(* Logix 5000 Rung export; software revision 16.03 *)

MODULES
   PDPMV1_60 : vendor None type None code None
   Local : vendor None type None code None
END_MODULES

TYPE PDPMV1_ModuleDef :   // Main module definition
STRUCT
   Output : SINT[1536];   // Output data
   Input : SINT[1536];   // Input data
   BP : PDPMV1_backplane2;   // Backplane status
   Status : PDPMV1_Status;   // Module status information
   MailboxCommand : PDPMV1_Command;   // Mailbox Command
   Mailbox : PDPMV1_Mailbox;   // Mailbox tags for optional applications
   CRC : PDPMV1_CRC_Struct;   // CRC status
   MailboxControl : PDPMV1_MBControl;   // Mailbox Control
   Util : PDPMV1_Util;   // Internal tags used for ladder logic processing. User applications should not overwrite any Util tags
END_STRUCT
END_TYPE

TYPE PDPMV1_Class1AcyclicRead_In :   // DPV1 acyclic read mailbox response
STRUCT
   ByteCount : INT;   // Byte count data block
   SlotNumber : SINT;   // Used in the slave to address the desired data block.
   SlaveAddress : SINT;   // Destination of slave (1-125)
   Length : SINT;   // Specifies the number of bytes of the data block to read
   Index : SINT;   // Index block
   ErrorDecode : SINT;   // If other than 0, refer to user manual for code information
   ErrorCode2 : SINT;   // If other than 0, refer to user manual for code information
   ErrorCode1 : SINT;   // If other than 0, refer to user manual for code information
   ExtendedFaultInfo : SINT;   // If other than 0, refer to user manual for code information
   FaultInformation : SINT;   // If other than 0, refer to user manual for code information
   Data : SINT[300];   // Returned data [1...n] array
END_STRUCT
END_TYPE

TYPE PDPMV1_GetSlaveConfig_In :   // GetSlaveConfig mailbox response
STRUCT
   ByteCount : INT;   // Byte count data block
   WordCount : INT;   // Word count data block
   SlaveAddress : INT;   // Destination of slave (1-125)
   ErrorCode : INT[1];   // If other than 0, refer to user manual for code information
   ReturnCode : INT;   // If other than 0, refer to user manual for code information
   FaultInformation : INT;   // If other than 0, refer to user manual for code information
   Identifier : SINT[245];   // Configuration from a specific connected PROFIBUS slave
END_STRUCT
END_TYPE

TYPE PDPMV1_backplane :   // This object stores variables used by the sample ladder for handshaking.
STRUCT
   Read : INT;   // Backplane read statistics
   Write : INT;   // Backplane write statistics
   Error : INT;   // Backplane error statistics
   LastRead : INT;   // Last read block index received from the module
   LastWrite : INT;   // Last write block index received from the module
   BlockIndex : INT;   // Block index of each copy of PROFIBUS input and output blocks
END_STRUCT
END_TYPE

TYPE PDPMV1_Status :   // Status block 0 or -1 for the MVI56-PDPMV1 module
STRUCT
   Pattern : SINT[12];   // Module indentification code
   Input_Size : INT;   // Input data size
   Output_Size : INT;   // Output data size
   Reserved_16 : INT;   // Reserved
   Reserved_18 : INT;   // Reserved
   Reserved_20 : INT;   // Reserved
   Input_Swap : SINT;   // User configured flag to indicate if input data is swapped before placing in the input image of the controller
   Output_Swap : SINT;   // User configured flag to indicate if output data is swapped before placing in the output image of the controller
   Module_Major_Ver : SINT;   // Module software major version number
   Module_Minor_Ver : SINT;   // Module software minor version number
   Fieldbus : PDPMV1_Fieldbus;   // PROFIBUS network status information
   Control : PDPMV1_Control;   // Module information
   Profibus_CRC32 : DINT;   // Profibus CRC32 value
   Module_CRC32 : DINT;   // Module CRC32 value
   Module : PDPMV1_Module;   // General module status to monitor data, mailbox and alarm exchange between the processor and the module
   Backplane : PDPMV1_backplane;   // Backplane status information
   Other : PDPMV1_other_status;   // General mailbox and cfg error information
END_STRUCT
END_TYPE

TYPE PDPMV1_Control :   // Control status
STRUCT
   serial_number : SINT[4];   // Module serial number
   version_MSB : SINT;   // Module version number (most significant byte)
   version_LSB : SINT;   // Module version number (least significant byte)
   mod_status_MSB : SINT;   // Module status (most significant byte)
   mod_status_LSB : SINT;   // Module status (least significant byte)
END_STRUCT
END_TYPE

TYPE PDPMV1_CRC_Struct :   // Module CRC structures
STRUCT
   In : PDPMV1_CRC;   // Mailbox response
   Out : PDPMV1_CRC;   // Mailbox request
END_STRUCT
END_TYPE

TYPE PDPMV1_Util :
STRUCT
   ByteSwapUtil : INT;   // Used for byte swap logic
   TempInt : INT;   // Used for integer formatting
   UtilCount : INT;   // Used for util count range
   Finishmailboxreading : BOOL;   // Used to finish mailbox requests and response reading
   TempInt2 : INT;   // Used to copy value to it then use it for comparison
   SetSlaveAddress101 : BOOL;   // Change the slave's PROFIBUS address 101 (only if slave supports this feature)
   SetSlaveAddress102 : BOOL;   // Change the slave's PROFIBUS address 102 (only if slave supports this feature)
   Class1AcyclicWrite101 : BOOL;   // Request the module to send acyclic write message to the slave
   Class1AcyclicWrite102 : BOOL;   // Request the module to send acyclic write message to the slave
   Class2AcyclicWrite101 : BOOL;   // Request the module to send Class2 acyclic write message to slave 101
   Class2AcyclicWrite102 : BOOL;   // Request the module to send Class2 acyclic write message to slave 102
   Finishgetlivelist : BOOL;   // Finish requesting the Live List information from the module
   FinishgetSlaveconfig : BOOL;   // Finish requesting configuration information from a slave
   FinishgetSlaveDiagnost : BOOL;   // Finish requesting slave diagnostics from a slave
   FinishSetSlaveAddr : BOOL;   // Finish changing the slaves PROFIBUS addressing
   FinishClass1AcyclicRead : BOOL;   // Finish requesting the module to send acyclic read message to slave
   FinishClass1AcyclicWrite : BOOL;   // Finish requesting the module to send acyclic write message to slave
   FinishStartStopSlaves : BOOL;   // Finish PROFIBUS communications with one or more slaves if supported
   FinishClass2AcyclicRead : BOOL;   // Finish requesting the module to send Class 2 acyclic read message to slave
   FinishClass2AcyclicWrite : BOOL;   // Finish requesting the module to send acyclic write message to slave
END_STRUCT
END_TYPE

TYPE PDPMV1_Class1AcyclicWrite_Out :   // DPV1 acyclic write mailbox request
STRUCT
   SlotNumber : SINT;   // Used in the slave to address the desired data block.
   SlaveAddress : SINT;   // Destination of slave (1-125)
   DataSize : INT;   // Object data size
   Length : SINT;   // Specifies the number of bytes of the data block to read
   Index : SINT;   // Index Block
   Data : SINT[300];   // Data that should be written [1...n]
END_STRUCT
END_TYPE

TYPE PDPMV1_AbortConnection_out :
STRUCT
   C_REF : INT;   // Connection reference that shall be terminated
   ReasonCode : SINT;   // Indicates the reason for the abort request. Value is user-specific. Range 0...15.
   Subnet : SINT;   // This parameter encodes information about the origin of the abort initiator. 0: No 1: Local 2: Remote
END_STRUCT
END_TYPE

TYPE PDPMV1_Class1AcyclicWrite_In :   // DPV1 acyclic write mailbox response
STRUCT
   ByteCount : INT;   // Byte count data block
   SlotNumber : SINT;   // Used in the slave to address the desired data block.
   SlaveAddress : SINT;   // Destination of slave (1-125)
   Length : SINT;   // Specifies the number of bytes of the data block to read
   Index : SINT;   // Index block
   ErrorDecode : SINT;   // If other than 0, refer to user manual for code information
   ErrorCode2 : SINT;   // If other than 0, refer to user manual for code information
   ErrorCode1 : SINT;   // If other than 0, refer to user manual for code information
   ExtendedFaultInfo : INT;   // If other than 0, refer to user manual for code information
   FaultInformation : INT;   // If other than 0, refer to user manual for code information
   Data : SINT[300];   // Returned data [1...n] array
END_STRUCT
END_TYPE

TYPE PDPMV1_GetSlaveConfig :   // GetSlaveConfig mailobox to retrieve configuration data from specific PROFIBUS slaves
STRUCT
   Out : PDPMV1_GetSlaveConfig_Out;   // mailbox request
   In : PDPMV1_GetSlaveConfig_In;   // mailbox response
END_STRUCT
END_TYPE

TYPE PDPMV1_Class2AcyclicRead_In :
STRUCT
   DataSize : INT;   // Byte count data block
   C_REF : INT;   // Connections references used to identify the connection later on. Range: 1-128
   Index : SINT;   // Index block
   SlotNumber : SINT;   // Used in the slave to address the desired data block.
   Length : INT;   // Specifies the number of bytes of the data block to read
   ErrorDecode : INT;   // If other than 0, refer to user manual for code information
   ErrorCode2 : SINT;   // If other than 0, refer to user manual for code information
   ErrorCode1 : SINT;   // If other than 0, refer to user manual for code information
   ExtendedFaultInfo : SINT;   // If other than 0, refer to user manual for code information
   FaultInformation : SINT;   // If other than 0, refer to user manual for code information
   Data : SINT[244];   // Returned data [1...n] array
END_STRUCT
END_TYPE

TYPE PDPMV1_Class2AcyclicWrite_In :   // DPV1 acyclic write mailbox response
STRUCT
   ByteCount : INT;   // Byte count data block
   C_REF : INT;   // Connection reference that shall be Read
   Index : SINT;   // Index block
   SlotNumber : SINT;   // Used in the slave to address the desired data block.
   Length : SINT;   // Specifies the number of bytes of the data block to read
   ErrorDecode : SINT;   // If other than 0, refer to user manual for code information
   ErrorCode2 : SINT;   // If other than 0, refer to user manual for code information
   ErrorCode1 : SINT;   // If other than 0, refer to user manual for code information
   ExtendedFaultInfo : SINT;   // If other than 0, refer to user manual for code information
   FaultInformation : SINT;   // If other than 0, refer to user manual for code information
   Data : SINT[244];   // Returned data [1...n] array
END_STRUCT
END_TYPE

TYPE PDPMV1_Module :   // Status data
STRUCT
   Mod_scan_count : INT;   // Incremented every module scan loop
   Mod_output_update : INT;   // Incremented at every output scan
   Mod_input_update : INT;   // Incremented at every input scan
   Mod_out_MB : INT;   // Incremented at every output mailbox processing
   Mod_in_MB : INT;   // Incremented at every intput mailbox processing
   Mod_alarm_ind : INT;   // Incremented at every alarm indication
   Mod_alarm_con : INT;   // Incremented at every alarm confirmation
   Reserved1 : INT;   // Reserved
   Reserved2 : INT;   // Reserved
END_STRUCT
END_TYPE

TYPE PDPMV1_Class1AcyclicRead :   // DPV1 acyclic read mailbox data structure
STRUCT
   Out : PDPMV1_Class1AcyclicRead_Out;   // Mailbox request
   In : PDPMV1_Class1AcyclicRead_In;   // Mailbox response
END_STRUCT
END_TYPE

TYPE PDPMV1_SetSlaveMode :   // SetSlaveMode mailbox that allows the processor to change the slave mode to interrupt input or output data update
STRUCT
   Out : PDPMV1_SetSlaveMode_Out;   // Mailbox Request
   In : PDPMV1_SetSlaveMode_In;   // Mailbox Response
END_STRUCT
END_TYPE

TYPE PDPMV1_GetSlaveDiagnostics_In :   // GetSlaveDiagnostics mailbox response
STRUCT
   RequestType : SINT;   // Type of request. 0 to use module memory RAM or 1 for live PROFIBUS network.
   SlaveAddress : SINT;   // Destination of slave (Range 1-125)
   ExtendedFaultInfo : INT;   // If other than 0, refer to user manual for code information
   FaultInformation : INT;   // If other than 0, refer to user manual for code information
   StationStatus1_2 : INT;   // Status of station types 1 and 2
   StationStatus3_4 : INT;   // Status of station types 3 and 4
   IdentNumber : INT;   // Unique ID assigned by the PROFIBUS User Organization
   ExtendedDiagnosticData : INT[200];   // Slave user-specific data. Refer to actual slave documentation for info
END_STRUCT
END_TYPE

TYPE PDPMV1_backplane2 :   // This object stores variables used by the sample ladder for handshaking.
STRUCT
   LastRead : INT;   // Last read block index received from the module
   LastWrite : INT;   // Last write block index received from the module
   BlockIndex : INT;   // Block index of each copy of PROFIBUS input and output blocks
END_STRUCT
END_TYPE

TYPE PDPMV1_Command :   // This object contains the command bits that request mailbox messages from the module.
STRUCT
   StopMode : BOOL;   // Set the module to stop mode (PROFIBUS communication is interrupted in stop mode)
   OperateMode : BOOL;   // Set the module to operate mode (module only communicates through PROFIBUS)
   ClearMode : BOOL;   // Set the module to clear mode (outputs are disabled)
   SynchCRC : BOOL;   // CRC synchronization
   GetLiveList : BOOL;   // Request the Live List information from the module
   GetSlaveConfig : BOOL;   // Request configuration information from slave
   SetSlaveMode : BOOL;   // Set the module to stop mode (PROFIBUS communication is interrupted in stop mode)
   GetSlaveDiagnostics : BOOL;   // Requests slave diagnostics from a slave
   SetSlaveAddress : BOOL;   // Change the slave's PROFIBUS address 100 (only if slave supports this feature)
   StartSlaves : BOOL;   // Restarts PROFIBUS communication with one or more slaves after a "StopSlave" mailbox
   StopSlaves : BOOL;   // Stop PROFIBUS communication with one or more slaves
   Class1AcyclicRead : BOOL;   // Request the module to send acyclic read message to slave
   Class1AcyclicWrite : BOOL;   // Request the module to send acyclic write message to the slave
   InitiateConnection : BOOL;   // Request to establish connection with a V1 slave that can handle class 2 messages
   AbortConnection : BOOL;   // Request to Abort an already established connection with a V1 slave that can handle class 2 messages
   Class2AcyclicRead : BOOL;   // Request the module to send class 2 acyclic Read message to a V1 slave
   Class2AcyclicWrite : BOOL;   // Request the module to send class 2 acyclic Write message to a V1 slave
END_STRUCT
END_TYPE

TYPE PDPMV1_SetSlaveMode_Out :   // Mailbox Request
STRUCT
   GroupSelect : SINT;   // Range 01h to FFh (Bit Coded). This parameter determines which group to address. Refer to the user manual for examples
   SlaveAddress : SINT;   // Range 1 to 125; 127 (Multicast address).
   ControlCommand : PDPMV1_ControlCommand;   // This parameter specifies the command to send (Unsync/Sync and Unfreeze/Freeze).
END_STRUCT
END_TYPE

TYPE PDPMV1_Fieldbus :   // Fieldbus status
STRUCT
   FB_Slave_Cfg_List : SINT[16];   // Bitmap structure containing PROFIBUS slave configuration (bit x = 1 means slave x is configured)
   FB_Slave_Data_xfer : SINT[16];   // Bitmap structure containing PROFIBUS slave data exchange status (bit x = 1 means slave x is transferring data to the module)
   FB_Slave_Diag : SINT[16];   // Bitmap structure containing PROFIBUS slave diagnostic info (bit x = 1 means slave x is reporting diagnostics)
   FB_Pad_Byte : SINT;   // Reserved
   FB_op_state : SINT;   // Operation state ( 00 = offline, 40 = stop, 80 = clear, C0= operate)
   FB_ident_MSB : SINT;   // Master identification code (most significant byte)
   FB_ident_LSB : SINT;   // Master identification code (least significant byte)
END_STRUCT
END_TYPE

TYPE PDPMV1_InitiateConnection_out :
STRUCT
   SlaveAddress : INT;   // Address of the slave to which a connection shall be established. Range: 0...126
   C_REF : INT;   // Connections references used to identify the connection later on. Range: 1-128
END_STRUCT
END_TYPE

TYPE PDPMV1_SetSlaveMode_In :   // Mailbox response
STRUCT
   GroupSelect : SINT;   // Range 01h to FFh (Bit Coded). This parameter determines which group to address. Refer to the user manual for examples
   SlaveAddress : SINT;   // Range 1 to 125; 127 (Multicast address).
   ControlCommand : PDPMV1_ControlCommand;   // This parameter specifies the command to send (Unsync/Sync and Unfreeze/Freeze).
   ExtendedFaultInfo : INT;   // If other than 0, refer to user manual for code information
   FaultInformation : INT;   // If other than 0, refer to user manual for code information
END_STRUCT
END_TYPE

TYPE PDPMV1_GetSlaveDiagnostics_Out :   // GetSlaveDiagnostics mailbox request
STRUCT
   RequestType : SINT;   // Type of request. 0 to use module memory RAM or 1 for live PROFIBUS network.
   SlaveAddress : SINT;   // Destination of slave (Range 1-125)
END_STRUCT
END_TYPE

TYPE PDPMV1_Class1AcyclicRead_Out :   // DPV1 acyclic read mailbox request
STRUCT
   SlotNumber : SINT;   // Used in the slave to address the desired data block.
   SlaveAddress : SINT;   // Destination of slave (1-125)
   DataSize : INT;   // Object data size
   Length : SINT;   // Specifies the number of bytes of the data block to read
   Index : SINT;   // Index block
END_STRUCT
END_TYPE

TYPE PDPMV1_Start_Stop_Slaves_Out :   // Mailbox request
STRUCT
   SlaveNumber : SINT[126];   // Slave number designation (1-125)
END_STRUCT
END_TYPE

TYPE PDPMV1_SetSlaveAddress :   // SetSlaveAddress mailbox that allows the module to dynamically change a PRIDUBUS address (only for slaves that supports it)
STRUCT
   Out : PDPMV1_SetSlaveAddress_Out;   // Mailbox request
   In : PDPMV1_SetSlaveAddress_In;   // Mailbox response
END_STRUCT
END_TYPE

TYPE PDPMV1_GetSlaveDiagnostics :   // GetSlaveDiagnostics mailbox to retrieve diagnostic information from specific PROFIBUS slaves
STRUCT
   Out : PDPMV1_GetSlaveDiagnostics_Out;   // Mailbox request
   In : PDPMV1_GetSlaveDiagnostics_In;   // Mailbox response
END_STRUCT
END_TYPE

TYPE PDPMV1_ControlCommand :   // Option bits for SetSlaveMode mailbox
STRUCT
   Reserved1 : BOOL;   // Reserved
   Reserved2 : BOOL;   // Reserved
   Unfreeze_Input : BOOL;   // Freeze mode is concluded when initiated
   Freeze_Input : BOOL;   // Causes the addressed slave to assume freeze mode.
   Unsynchronize_Output : BOOL;   // Unsynchronized output data
   Synchronize_Output : BOOL;   // Synchronized output data
   Reserved3 : BOOL[32];   // Reserved
END_STRUCT
END_TYPE

TYPE PDPMV1_Mailbox :   // Stores all mailbox request and response registers
STRUCT
   GetLiveList : PDPMV1_GetLiveList;   // Gets information from all nodes on the network
   GetSlaveConfig : PDPMV1_GetSlaveConfig;   // Get slave configuration
   SetSlaveMode : PDPMV1_SetSlaveMode;   // Send special control command to one or several slaves (Sync/Freeze)
   GetSlaveDiagnostics : PDPMV1_GetSlaveDiagnostics;   // Get diagnostic information from a slave
   SetSlaveAddress : PDPMV1_SetSlaveAddress;   // Set node address of a slave (if supported by the slave)
   StartStopSlaves : PDPMV1_Start_Stop_Slaves;   // Start/Stop slaves dynamically
   Class1AcyclicRead : PDPMV1_Class1AcyclicRead;   // Initiates a DPV1 class 1 acyclic read request.
   Class1AcyclicWrite : PDPMV1_Class1AcyclicWrite;   // Initiates a DPV1 class 1 acyclic write request.
   Alarm : PDPMV1_Alarm;   // Alarm message transferred by a slave to the master
   InitiateConnection : PDPMV1_InitiateConnection;   // mailbox form used to initiate connection with v1 slave before sending class2 messages.
   AbortConnection : PDPMV1_AbortConnection;   // mailbox form used to abort an already established connection with v1 slave before sending class2 messages.
   Class2AcyclicRead : PDPMV1_Class2AcyclicRead;   // mailbox form used to send a class 2 messages to read acyclic data
   Class2AcyclicWrite : PDPMV1_Class2AcyclicWrite;   // mailbox form used to send a class 2 messages to write acyclic data
END_STRUCT
END_TYPE

TYPE PDPMV1_Alarm :   // DPV1 alarm data received by the module
STRUCT
   ByteCount : INT;   // Byte count data block
   SlotNumber : SINT;   // Used in the slave to address the desired data block. Range 0-254
   SlaveAddress : SINT;   // Destination of slave (1-125)
   AlarmSpecAck : SINT;   // Additional alarm information
   SeqNumber : SINT;   // Unique ID number of the alarm. Range 0-31.
   ExtDiag : SINT;   // Extended Diagnostic Flag (FFh - flag set and 00h - flag cleared).
   AlarmType : SINT;   // Identifies alarm type. Range is from 1 to 6, 32 to 126.
   FaultInformation : SINT;   // If other than 0, refer to user manual for code information
   Data : SINT[500];   // Returned data [1...n] array with additional manf. spec alarm info.
END_STRUCT
END_TYPE

TYPE PDPMV1_GetSlaveConfig_Out :   // GetSlaveConfig mailbox request
STRUCT
   SlaveAddress : INT;   // Destination of slave (1-125)
END_STRUCT
END_TYPE

TYPE PDPMV1_Class2AcyclicRead_Out :
STRUCT
   C_REF : INT;   // Connection reference that shall be terminated
   Index : SINT;   // Used in the slave for addressing of the desired data block. Range 0...254
   SlotNumber : SINT;   // Used in the slave for addressing of the desired data block. Range 0...254
   Length : INT;   // Number of bytes to write
END_STRUCT
END_TYPE

TYPE PDPMV1_GetLiveList :   // GetLiveList mailbox to retrieve the live list information from PROFIBUS network, informing the slaves that are communicating
STRUCT
   ReturnCode : SINT;   // Returned code about the nodes on the network
   FaultInfo : SINT;   // If other than 0, refer to user manual for code information
   Station : SINT[127];   // Station type contents.
END_STRUCT
END_TYPE

TYPE PDPMV1_AbortConnection_In :
STRUCT
   C_REF : INT;   // Connection reference that shall be terminated.
   ReasonCode : SINT;   // Indicates the reason for the abort request. Value is user-specific. Range 0...15
   Subnet : SINT;   // This parameter encodes information about the origin of the abort initiator. 0: No 1: Local 2: Remote 3...255: (reserved)
   ExtendedFaultInformation : INT;   // If ‘Fault Information’ equals 000Ah or 000Bh, additional information of the error can be found here. For more information,
   FaultInformation : INT;   // If ‘Invalid Other’ is returned in the Message Information word in the header of the response,
END_STRUCT
END_TYPE

TYPE PDPMV1_CRC :   // This object stores CRC values for both Profibus and the module.
STRUCT
   ProfibusCRC : DINT;   // Stores Profibus CRC32 values
   ModuleCRC : DINT;   // Stores Module CRC32 values
END_STRUCT
END_TYPE

TYPE PDPMV1_SetSlaveAddress_Out :   // Mailbox request
STRUCT
   ByteCount : INT;   // Byte count data block
   NewSlaveAddress : SINT;   // Range 1 to 125, specifies the new address of the slave
   CurrentSlaveAddress : SINT;   // Range 1 to 125, specifies the current address of the slave
   SlaveIdentNumber : INT;   // Indent number for the slave
   No_add_Chg : INT;   // specifies whether it is allowed to change the slave address again later
   MessageDataByte : SINT[400];   // Message data byte array for user-specific data
END_STRUCT
END_TYPE

TYPE PDPMV1_InitiateConnection :
STRUCT
   Out : PDPMV1_InitiateConnection_out;   // Mailbox Request
   In : PDPMV1_InitiateConnection_In;   // Mailbox response
END_STRUCT
END_TYPE

TYPE PDPMV1_Class2AcyclicWrite_Out :   // DPV1 acyclic write mailbox request
STRUCT
   DataSize : INT;   // Object data size
   C_REF : INT;   // Connection reference that shall be terminated
   Index : SINT;   // Index block
   SlotNumber : SINT;   // Used in the slave to address the desired data block.
   Length : INT;   // Specifies the number of bytes of the data block to read
   Data : SINT[244];   // Data that should be written [1...n]
END_STRUCT
END_TYPE

TYPE PDPMV1_other_status :   // This object contains specific information, such as the number of mailbox and alarms located in the mailbox queue.
STRUCT
   Cfg_file_error : INT;   // Bit0 = PDPMV1.CFG, Bit 1 = WATTCP.CFG, Bit 2 = PDPMV1.DDB, Bit3=PDPMV1.XML
   R_120 : INT;   // Not Used
   R_122 : INT;   // Not Used
   R_124 : INT;   // Not Used
   R_126 : INT;   // Not Used
   R_128 : INT;   // Not Used
   R_130 : INT;   // Not Used
   R_132 : INT;   // Not Used
   R_134 : INT;   // Not Used
   R_136 : INT;   // Not Used
   R_138 : INT;   // Not Used
   R_140 : INT;   // Not Used
   R_142 : INT;   // Not Used
   R_144 : INT;   // Not Used
   In_MB_queue : INT;   // Number of messages in the input mailbox queue
   Out_MB_queue : INT;   // Number of messages in the output mailbox queue
   Alarm_MB_queue : INT;   // Number of messages in the alarm mailbox queue
   Last_out_MB : INT;   // Number of messages in the output mailbox queue
   Cur_in_MB : INT;   // Number of messages currently in the input mailbox queue
   Cur_alarm_MB : INT;   // Number of messages currently in the alarm mailbox queue
END_STRUCT
END_TYPE

TYPE PDPMV1_Class2AcyclicWrite :   // DPV1 acyclic write mailbox data structure
STRUCT
   Out : PDPMV1_Class2AcyclicWrite_Out;   // Mailbox request
   In : PDPMV1_Class2AcyclicWrite_In;   // Mailbox response
END_STRUCT
END_TYPE

TYPE PDPMV1_Start_Stop_Slaves :   // Start/Stop Slaves mailbox allows the processor to restart or hault slave communication.
STRUCT
   Out : PDPMV1_Start_Stop_Slaves_Out;   // Mailbox Request
   In : PDPMV1_Start_Stop_Slaves_In;   // Mailbox Response
END_STRUCT
END_TYPE

TYPE PDPMV1_Class1AcyclicWrite :   // DPV1 acyclic write mailbox data structure
STRUCT
   Out : PDPMV1_Class1AcyclicWrite_Out;   // Mailbox request
   In : PDPMV1_Class1AcyclicWrite_In;   // Mailbox response
END_STRUCT
END_TYPE

TYPE PDPMV1_Class2AcyclicRead :
STRUCT
   Out : PDPMV1_Class2AcyclicRead_Out;   // Mailbox request
   In : PDPMV1_Class2AcyclicRead_In;   // Mailbox response
END_STRUCT
END_TYPE

TYPE PDPMV1_MBControl :   // PDPMV1 Mailbox Control status.
STRUCT
   Out_MB_index : INT;   // Reserved
   In_MB_index : INT;   // Reserved
   Alarm_MB_index : INT;   // Reserved
   In_Last_Out_MB : INT;   // Last out mailbox message ID processed from output image
   In_Last_In_MB : INT;   // Current in mailbox control index
   In_Last_Alarm_MB : INT;   // Current alarm control index
   Out_Last_Out_MB : INT;   // Reserved
   Out_Last_In_MB : INT;   // Reserved
   Out_Last_Alarm_MB : INT;   // Reserved
END_STRUCT
END_TYPE

TYPE PDPMV1_AbortConnection :
STRUCT
   Out : PDPMV1_AbortConnection_out;   // Mailbox Request
   In : PDPMV1_AbortConnection_In;   // Mailbox Response
END_STRUCT
END_TYPE

TYPE PDPMV1_SetSlaveAddress_In :   // Mailbox response
STRUCT
   ByteCount : INT;   // Byte count data block
   NewSlaveAddress : SINT;   // Range 1 to 125, specifies the new address of the slave
   CurrentSlaveAddress : SINT;   // Range 1 to 125, specifies the current address of the slave
   SlaveIdentNumber : INT;   // Indent number for the slave
   No_add_Chg : INT;   // specifies whether it is allowed to change the slave address again later
   ErrorCode1_2 : INT;   // If other than 0, refer to user manual for code information
   ErrorCode3_4 : INT;   // If other than 0, refer to user manual for code information
   ReturnCode : INT;   // If other than 0, refer to user manual for code information
   FaultInformation : INT;   // If other than 0, refer to user manual for code information
   MessageDataByte : SINT[400];   // Message data byte array for user-specific data
END_STRUCT
END_TYPE

TYPE PDPMV1_Start_Stop_Slaves_In :   // Mailbox response
STRUCT
   AdditionalFaultInfo : INT;   // If other than 0, refer to user manual for code information
   FaultInformation : INT;   // If other than 0, refer to user manual for code information
   SlaveNumber : SINT[126];   // Slave number designation (Range 1-125)
END_STRUCT
END_TYPE

TYPE PDPMV1_InitiateConnection_In :   // This tag holds the response parameters after the user sends mailbox to initiate connection with V1 slave
STRUCT
   SizeofdatainBytes : INT;   // Size of data being read
   C_REF : INT;   // Connections references used to identify the connection later on. Range: 1-128
   MaxDataLength : SINT;   // The slave’s maximum data length in bytes (reported by the slave in DP Initiate.res).
   SlaveAddress : SINT;   // Address of the slave to which a connection shall be established. Range: 0...126
   MinmumSlaveTimeout : INT;   // The minimum slave timeout value supported by the slave (in multiples of 10ms).
   ErrorDecode : SINT;   // If ‘Fault Information’ equals 0010h, additional information according to the DPV1 specification
   ErrorCode2 : SINT;   // If ‘Fault Information’ equals 0010h, additional information according to the DPV1 specification
   ErrorCode1 : SINT;   // If ‘Fault Information’ equals 0010h, additional information according to the DPV1 specification
   ExtendedFaultInformation : INT;   // If ‘Fault Information’ equals 000Ah or 000Bh, additional information of the error can be found here. For more information, see
   FaultInformation : INT;   // If ‘Invalid Other’ is returned in the Message Information word in the header of the response, information about the fault
   SendTimeout : INT;   // Defines the control time (timebase 10ms) for the supervision of the connection between the slave and the master. Range 6...655
   FeatureSupported2 : SINT;   // (reserved for future use)
   FeatureSupported1 : SINT;   // Identifies the supported C2-service functionality as follows: b0: DPV1_RW. This bit is set if the services C2_Read and C2_Write
   ProfileFeatures2 : SINT;   // Identifies the supported service functionality regarding the used profile definition. The meaning of these registers are profil
   ProfileFeatures1 : SINT;   // Identifies the supported service functionality regarding the used profile definition. The meaning of these registers are profil
   ProfileIdentNumber : INT;   // This parameter identifies a unique profile definition. The Profile Ident Number is taken from the pool of Ident Numbers managed
   S_Length : SINT;   // This parameter specifies the length of the S_Address parameter (see table below). Default value is 02h.
   S_Type : SINT;   // This parameter indicates the presence of the optional Network/MAC address of the source. b0: 1: A Network/MAC address is presen
   D_Length : SINT;   // This value specifies the length of the D_Address parameter (see table below). Default value is 02h.
   D_Type : SINT;   // This parameter indicates the presence of the optional Network/MAC address of the destination. b0: 1: A Network/MAC address is p
   S_Address : INT;   // This field holds additional address information about the source. It’s structure depends on the settings in S_Type.
   D_Address : INT;   // This field holds additional address information about the destination. It’s structure depends on the settings in D_Type
END_STRUCT
END_TYPE

ADD_ON_INSTRUCTION AOI69PDPMV1_60   (* revision 1.4, vendor ProSoft Technology Inc. *)
// Add-On - MVI69-PDPMV1(Block size 60).
// Revision note:
// v1.4 - Added support for class 2 messages that was supported in a specific  V1 slaves.
VAR_IN_OUT
   Connection_Input : INT[62]; {required}   // Connection Input to be associated to the MVI69PDPMV1 Input Array
   Connection_Output : INT[61]; {required}   // Connection Output to be associated to the MVI69-PDPMV1 Output Array
   MVI69PDPMV1 : PDPMV1_ModuleDef; {required}
END_VAR

ROUTINE Logic   (* ladder *)
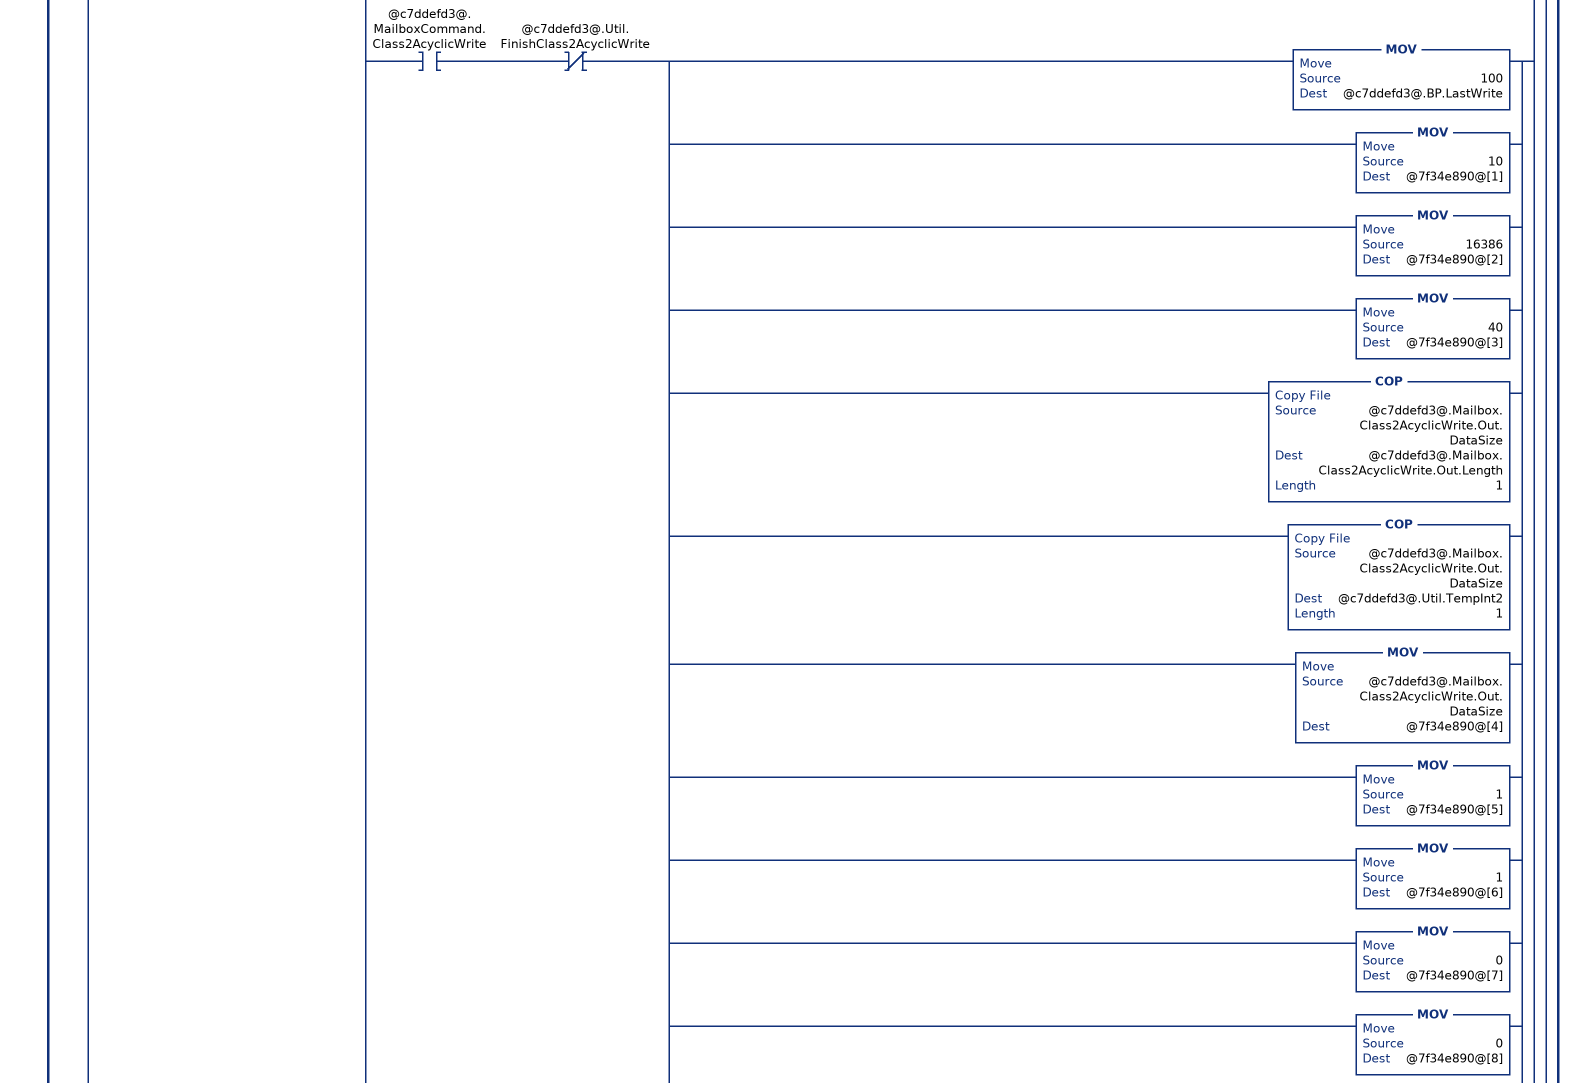
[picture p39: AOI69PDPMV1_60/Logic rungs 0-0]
   // This rung is used to verify if the module has sent a new input block to the processor. The trigger is when the input image offset 0 (Read Block ID) is different than the last one processed by the processor
   0: NEQ(@8b565331@[0],@c7ddefd3@.BP.LastRead)[MOV(@8b565331@[0],@c7ddefd3@.BP.LastRead) ,EQU(@c7ddefd3@.BP.LastRead,-1) [COP(@8b565331@[2],@c7ddefd3@.Status.Pattern[0],20) ,COP(@8b565331@[13],@c7ddefd3@.Status.Input_Swap,4) ,COP(@8b565331@[15],@c7ddefd3@.Status.Fieldbus.FB_Slave_Cfg_List[0],52) ,COP(@8b565331@[41],@c7ddefd3@.Status.Control.serial_number[0],8) ,COP(@8b565331@[45],@c7ddefd3@.Status.Profibus_CRC32,2) ] ,EQU(@c7ddefd3@.BP.LastRead,0) [COP(@8b565331@[2],@c7ddefd3@.Status.Module.Mod_scan_count,9) ,COP(@8b565331@[11],@c7ddefd3@.Status.Backplane.Read,3) ,COP(@8b565331@[14],@c7ddefd3@.Status.Other.Cfg_file_error,20) ] ,LIM(1,@c7ddefd3@.BP.LastRead,16) [LIM(1,@c7ddefd3@.BP.LastRead,15) [CPT(@c7ddefd3@.BP.BlockIndex,(@c7ddefd3@.BP.LastRead-1)*100) ,COP(@8b565331@[2],@c7ddefd3@.Input[@c7ddefd3@.BP.BlockIndex],100) ] ,EQU(@c7ddefd3@.BP.LastRead,16) COP(@8b565331@[2],@c7ddefd3@.Input[1500],36) ,COP(@8b565331@[52],@c7ddefd3@.MailboxControl.In_Last_Out_MB,2) ,COP(@8b565331@[56],@c7ddefd3@.CRC.In.ProfibusCRC,2) ] ,LIM(100,@c7ddefd3@.BP.LastRead,102) [EQU(100,@c7ddefd3@.BP.LastRead) LIM(0,@8b565331@[2],2) [OTU(@c7ddefd3@.MailboxCommand.StopMode) ,OTU(@c7ddefd3@.MailboxCommand.OperateMode) ,OTU(@c7ddefd3@.MailboxCommand.ClearMode) ,OTU(@c7ddefd3@.MailboxCommand.SetSlaveMode) ] ,XIC(@c7ddefd3@.Util.Finishgetlivelist) [EQU(@8b565331@[4],24) EQU(100,@c7ddefd3@.BP.LastRead) [MOV(@8b565331@[5],@c7ddefd3@.Util.UtilCount) ,COP(@8b565331@[18],@c7ddefd3@.Mailbox.GetLiveList.Station[0],88) ,LEQ(@c7ddefd3@.Util.UtilCount,88) OTU(@c7ddefd3@.Util.Finishgetlivelist) ] ,EQU(101,@c7ddefd3@.BP.LastRead) [COP(@8b565331@[2],@c7ddefd3@.Mailbox.GetLiveList.Station[88],39) ,OTU(@c7ddefd3@.Util.Finishgetlivelist) ] ] ,EQU(@8b565331@[4],3) [COP(@8b565331@[10],@c7ddefd3@.Mailbox.SetSlaveMode.In.GroupSelect,2) ,MOV(@8b565331@[11],@c7ddefd3@.Util.TempInt) ,SWPB(@c7ddefd3@.Util.TempInt,REVERSE,@c7ddefd3@.Util.ByteSwapUtil) ,COP(@c7ddefd3@.Util.ByteSwapUtil,@c7ddefd3@.Mailbox.SetSlaveMode.In.ControlCommand,1) ,MOV(@8b565331@[16],@c7ddefd3@.Mailbox.SetSlaveMode.In.ExtendedFaultInfo) ,MOV(@8b565331@[17],@c7ddefd3@.Mailbox.SetSlaveMode.In.FaultInformation) ] ,XIC(@c7ddefd3@.Util.FinishgetSlaveDiagnost) [EQU(100,@c7ddefd3@.BP.LastRead) EQU(@8b565331@[4],4) [MOV(@8b565331@[5],@c7ddefd3@.Util.UtilCount) ,COP(@8b565331@[10],@c7ddefd3@.Mailbox.GetSlaveDiagnostics.In.RequestType,2) ,MOV(@8b565331@[16],@c7ddefd3@.Mailbox.GetSlaveDiagnostics.In.ExtendedFaultInfo) ,MOV(@8b565331@[17],@c7ddefd3@.Mailbox.GetSlaveDiagnostics.In.FaultInformation) ,MOV(@8b565331@[18],@c7ddefd3@.Mailbox.GetSlaveDiagnostics.In.StationStatus1_2) ,MOV(@8b565331@[19],@c7ddefd3@.Mailbox.GetSlaveDiagnostics.In.StationStatus3_4) ,MOV(@8b565331@[20],@c7ddefd3@.Mailbox.GetSlaveDiagnostics.In.IdentNumber) ,COP(@8b565331@[21],@c7ddefd3@.Mailbox.GetSlaveDiagnostics.In.ExtendedDiagnosticData[0],41) ,LEQ(@c7ddefd3@.Util.UtilCount,41) OTU(@c7ddefd3@.Util.FinishgetSlaveDiagnost) ] ,EQU(101,@c7ddefd3@.BP.LastRead) [SUB(@c7ddefd3@.Util.UtilCount,41,@c7ddefd3@.Util.UtilCount) ,COP(@8b565331@[2],@c7ddefd3@.Mailbox.GetSlaveDiagnostics.In.ExtendedDiagnosticData[41],60) ,LEQ(@c7ddefd3@.Util.UtilCount,60) OTU(@c7ddefd3@.Util.FinishgetSlaveDiagnost) ] ,EQU(102,@c7ddefd3@.BP.LastRead) [COP(@8b565331@[2],@c7ddefd3@.Mailbox.GetSlaveDiagnostics.In.ExtendedDiagnosticData[101],24) ,OTU(@c7ddefd3@.Util.FinishgetSlaveDiagnost) ] ] ,XIC(@c7ddefd3@.Util.FinishgetSlaveconfig) [EQU(@c7ddefd3@.BP.LastRead,100) EQU(@8b565331@[4],5) [MOV(@8b565331@[5],@c7ddefd3@.Mailbox.GetSlaveConfig.In.ByteCount) ,MOV(@8b565331@[10],@c7ddefd3@.Util.ByteSwapUtil) ,SWPB(@c7ddefd3@.Util.ByteSwapUtil,REVERSE,@c7ddefd3@.Mailbox.GetSlaveConfig.In.SlaveAddress) ,COP(@8b565331@[14],@c7ddefd3@.Mailbox.GetSlaveConfig.In.ErrorCode[0],2) ,MOV(@8b565331@[16],@c7ddefd3@.Mailbox.GetSlaveConfig.In.ReturnCode) ,MOV(@8b565331@[17],@c7ddefd3@.Mailbox.GetSlaveConfig.In.FaultInformation) ,COP(@8b565331@[18],@c7ddefd3@.Mailbox.GetSlaveConfig.In.Identifier[0],88) ,LEQ(@c7ddefd3@.Mailbox.GetSlaveConfig.In.ByteCount,88) OTU(@c7ddefd3@.Util.FinishgetSlaveconfig) ] ,EQU(@c7ddefd3@.BP.LastRead,101) [SUB(@c7ddefd3@.Mailbox.GetSlaveConfig.In.ByteCount,88,@c7ddefd3@.Mailbox.GetSlaveConfig.In.ByteCount) ,COP(@8b565331@[2],@c7ddefd3@.Mailbox.GetSlaveConfig.In.Identifier[88],120) ,LEQ(@c7ddefd3@.Mailbox.GetSlaveConfig.In.ByteCount,120) OTU(@c7ddefd3@.Util.FinishgetSlaveconfig) ] ,EQU(@c7ddefd3@.BP.LastRead,102) [COP(@8b565331@[2],@c7ddefd3@.Mailbox.GetSlaveConfig.In.Identifier[208],48) ,OTU(@c7ddefd3@.Util.FinishgetSlaveconfig) ] ] ,XIC(@c7ddefd3@.Util.FinishSetSlaveAddr) [EQU(@8b565331@[4],6) EQU(@c7ddefd3@.BP.LastRead,100) [MOV(@8b565331@[5],@c7ddefd3@.Mailbox.SetSlaveAddress.In.ByteCount) ,COP(@8b565331@[10],@c7ddefd3@.Mailbox.SetSlaveAddress.In.NewSlaveAddress,2) ,MOV(@8b565331@[11],@c7ddefd3@.Mailbox.SetSlaveAddress.In.SlaveIdentNumber) ,MOV(@8b565331@[12],@c7ddefd3@.Util.ByteSwapUtil) ,SWPB(@c7ddefd3@.Util.ByteSwapUtil,REVERSE,@c7ddefd3@.Mailbox.SetSlaveAddress.In.No_add_Chg) ,MOV(@8b565331@[14],@c7ddefd3@.Mailbox.SetSlaveAddress.In.ErrorCode1_2) ,MOV(@8b565331@[15],@c7ddefd3@.Mailbox.SetSlaveAddress.In.ErrorCode3_4) ,MOV(@8b565331@[16],@c7ddefd3@.Mailbox.SetSlaveAddress.In.ReturnCode) ,MOV(@8b565331@[17],@c7ddefd3@.Mailbox.SetSlaveAddress.In.FaultInformation) ,COP(@8b565331@[18],@c7ddefd3@.Mailbox.SetSlaveAddress.In.MessageDataByte[0],88) ,LEQ(@c7ddefd3@.Mailbox.SetSlaveAddress.Out.ByteCount,88) OTU(@c7ddefd3@.Util.FinishSetSlaveAddr) ,GRT(@c7ddefd3@.Mailbox.SetSlaveAddress.Out.ByteCount,88) [SUB(88,@c7ddefd3@.Mailbox.SetSlaveAddress.Out.ByteCount,@c7ddefd3@.Mailbox.SetSlaveAddress.Out.ByteCount) ,OTL(@c7ddefd3@.Util.SetSlaveAddress101) ,OTL(@c7ddefd3@.Util.Finishmailboxreading) ] ] ,EQU(@c7ddefd3@.BP.LastRead,101) XIC(@c7ddefd3@.Util.Finishmailboxreading) [LEQ(@c7ddefd3@.Mailbox.SetSlaveAddress.Out.ByteCount,120) [COP(@8b565331@[2],@c7ddefd3@.Mailbox.SetSlaveAddress.In.MessageDataByte[88],120) ,OTU(@c7ddefd3@.Util.Finishmailboxreading) ,OTU(@c7ddefd3@.Util.SetSlaveAddress101) ,MOV(0,@c7ddefd3@.Mailbox.SetSlaveAddress.Out.ByteCount) ] ,GRT(@c7ddefd3@.Mailbox.SetSlaveAddress.Out.ByteCount,120) [SUB(120,@c7ddefd3@.Mailbox.SetSlaveAddress.Out.ByteCount,@c7ddefd3@.Mailbox.SetSlaveAddress.Out.ByteCount) ,OTL(@c7ddefd3@.Util.FinishSetSlaveAddr) ,OTL(@c7ddefd3@.Util.Finishmailboxreading) ] ] ,EQU(@c7ddefd3@.BP.LastRead,102) [COP(@8b565331@[2],@c7ddefd3@.Mailbox.SetSlaveAddress.In.MessageDataByte[208],48) ,OTU(@c7ddefd3@.Util.FinishSetSlaveAddr) ,OTU(@c7ddefd3@.Util.Finishmailboxreading) ,MOV(0,@c7ddefd3@.Mailbox.SetSlaveAddress.Out.ByteCount) ] ] ,XIC(@c7ddefd3@.Util.FinishStartStopSlaves) [LIM(11,@8b565331@[4],12) EQU(@c7ddefd3@.BP.LastRead,100) [MOV(@8b565331@[16],@c7ddefd3@.Mailbox.StartStopSlaves.In.AdditionalFaultInfo) ,MOV(@8b565331@[17],@c7ddefd3@.Mailbox.StartStopSlaves.In.FaultInformation) ,COP(@8b565331@[18],@c7ddefd3@.Mailbox.StartStopSlaves.In.SlaveNumber[0],88) ] ,EQU(@c7ddefd3@.BP.LastRead,101) [COP(@8b565331@[2],@c7ddefd3@.Mailbox.StartStopSlaves.In.SlaveNumber[88],40) ,OTU(@c7ddefd3@.Util.FinishStartStopSlaves) ] ] ,XIC(@c7ddefd3@.Util.FinishClass1AcyclicRead) [EQU(100,@c7ddefd3@.BP.LastRead) EQU(@8b565331@[4],32) [MOV(@8b565331@[5],@c7ddefd3@.Mailbox.Class1AcyclicRead.In.ByteCount) ,COP(@8b565331@[10],@c7ddefd3@.Mailbox.Class1AcyclicRead.In.SlotNumber,2) ,COP(@8b565331@[11],@c7ddefd3@.Mailbox.Class1AcyclicRead.In.Length,2) ,COP(@8b565331@[14],@c7ddefd3@.Mailbox.Class1AcyclicRead.In.ErrorDecode,1) ,COP(@8b565331@[15],@c7ddefd3@.Mailbox.Class1AcyclicRead.In.ErrorCode2,2) ,MOV(@8b565331@[16],@c7ddefd3@.Mailbox.Class1AcyclicRead.In.ExtendedFaultInfo) ,MOV(@8b565331@[17],@c7ddefd3@.Mailbox.Class1AcyclicRead.In.FaultInformation) ,COP(@8b565331@[18],@c7ddefd3@.Mailbox.Class1AcyclicRead.In.Data[0],88) ,LEQ(@c7ddefd3@.Mailbox.Class1AcyclicRead.In.ByteCount,88) OTU(@c7ddefd3@.Util.FinishClass1AcyclicRead) ] ,EQU(101,@c7ddefd3@.BP.LastRead) [SUB(@c7ddefd3@.Mailbox.Class1AcyclicRead.In.ByteCount,88,@c7ddefd3@.Mailbox.Class1AcyclicRead.In.ByteCount) ,COP(@8b565331@[2],@c7ddefd3@.Mailbox.Class1AcyclicRead.In.Data[88],120) ,LEQ(@c7ddefd3@.Mailbox.Class1AcyclicRead.In.ByteCount,120) OTU(@c7ddefd3@.Util.FinishClass1AcyclicRead) ] ,EQU(102,@c7ddefd3@.BP.LastRead) [COP(@8b565331@[2],@c7ddefd3@.Mailbox.Class1AcyclicRead.In.Data[208],48) ,OTU(@c7ddefd3@.Util.FinishClass1AcyclicRead) ] ] ,XIC(@c7ddefd3@.Util.FinishClass1AcyclicWrite) [EQU(100,@c7ddefd3@.BP.LastRead) EQU(@8b565331@[4],33) [MOV(@8b565331@[5],@c7ddefd3@.Mailbox.Class1AcyclicWrite.In.ByteCount) ,COP(@8b565331@[10],@c7ddefd3@.Mailbox.Class1AcyclicWrite.In.SlotNumber,2) ,COP(@8b565331@[11],@c7ddefd3@.Mailbox.Class1AcyclicWrite.In.Length,2) ,COP(@8b565331@[14],@c7ddefd3@.Mailbox.Class1AcyclicWrite.In.ErrorDecode,1) ,COP(@8b565331@[15],@c7ddefd3@.Mailbox.Class1AcyclicWrite.In.ErrorCode2,2) ,MOV(@8b565331@[16],@c7ddefd3@.Mailbox.Class1AcyclicWrite.In.ExtendedFaultInfo) ,MOV(@8b565331@[17],@c7ddefd3@.Mailbox.Class1AcyclicWrite.In.FaultInformation) ,COP(@8b565331@[18],@c7ddefd3@.Mailbox.Class1AcyclicWrite.In.Data[0],88) ,LEQ(@c7ddefd3@.Mailbox.Class1AcyclicWrite.In.ByteCount,88) OTU(@c7ddefd3@.Util.FinishClass1AcyclicWrite) ,GRT(@c7ddefd3@.Mailbox.Class1AcyclicWrite.In.ByteCount,88) OTL(@c7ddefd3@.Util.Finishmailboxreading) ] ,EQU(101,@c7ddefd3@.BP.LastRead) XIC(@c7ddefd3@.Util.Finishmailboxreading) [LES(@c7ddefd3@.Mailbox.Class1AcyclicWrite.In.ByteCount,120) [COP(@8b565331@[2],@c7ddefd3@.Mailbox.Class1AcyclicWrite.In.Data[88],@c7ddefd3@.Mailbox.Class1AcyclicWrite.In.ByteCount) ,OTU(@c7ddefd3@.Util.FinishClass1AcyclicWrite) ,OTU(@c7ddefd3@.Util.Finishmailboxreading) ,OTU(@c7ddefd3@.Util.Class1AcyclicWrite101) ] ,GRT(@c7ddefd3@.Mailbox.Class1AcyclicWrite.In.ByteCount,120) OTL(@c7ddefd3@.Util.Finishmailboxreading) ] ,EQU(102,@c7ddefd3@.BP.LastRead) XIC(@c7ddefd3@.Util.Finishmailboxreading) [COP(@8b565331@[2],@c7ddefd3@.Mailbox.Class1AcyclicWrite.In.Data[208],48) ,OTU(@c7ddefd3@.Util.FinishClass1AcyclicWrite) ,OTU(@c7ddefd3@.Util.Finishmailboxreading) ] ] ,EQU(@8b565331@[4],37) [MOV(@8b565331@[5],@c7ddefd3@.Mailbox.InitiateConnection.In.SizeofdatainBytes) ,MOV(@8b565331@[10],@c7ddefd3@.Mailbox.InitiateConnection.In.C_REF) ,COP(@8b565331@[11],@c7ddefd3@.Mailbox.InitiateConnection.In.MaxDataLength,2) ,MOV(@8b565331@[12],@c7ddefd3@.Mailbox.InitiateConnection.In.MinmumSlaveTimeout) ,COP(@8b565331@[14],@c7ddefd3@.Mailbox.InitiateConnection.In.ErrorDecode,1) ,COP(@8b565331@[15],@c7ddefd3@.Mailbox.InitiateConnection.In.ErrorCode2,2) ,MOV(@8b565331@[16],@c7ddefd3@.Mailbox.InitiateConnection.In.ExtendedFaultInformation) ,MOV(@8b565331@[17],@c7ddefd3@.Mailbox.InitiateConnection.In.FaultInformation) ,MOV(@8b565331@[18],@c7ddefd3@.Mailbox.InitiateConnection.In.SendTimeout) ,COP(@8b565331@[19],@c7ddefd3@.Mailbox.InitiateConnection.In.FeatureSupported2,2) ,COP(@8b565331@[20],@c7ddefd3@.Mailbox.InitiateConnection.In.ProfileFeatures2,2) ,MOV(@8b565331@[21],@c7ddefd3@.Mailbox.InitiateConnection.In.ProfileIdentNumber) ,COP(@8b565331@[22],@c7ddefd3@.Mailbox.InitiateConnection.In.S_Length,2) ,COP(@8b565331@[23],@c7ddefd3@.Mailbox.InitiateConnection.In.D_Length,2) ,MOV(@8b565331@[24],@c7ddefd3@.Mailbox.InitiateConnection.In.S_Address) ,MOV(@8b565331@[25],@c7ddefd3@.Mailbox.InitiateConnection.In.D_Address) ] ,EQU(@8b565331@[4],38) [MOV(@8b565331@[10],@c7ddefd3@.Mailbox.AbortConnection.In.C_REF) ,COP(@8b565331@[11],@c7ddefd3@.Mailbox.AbortConnection.In.ReasonCode,2) ,MOV(@8b565331@[16],@c7ddefd3@.Mailbox.AbortConnection.In.ExtendedFaultInformation) ,MOV(@8b565331@[17],@c7ddefd3@.Mailbox.AbortConnection.In.FaultInformation) ] ,XIC(@c7ddefd3@.Util.FinishClass2AcyclicRead) [EQU(100,@c7ddefd3@.BP.LastRead) EQU(@8b565331@[4],39) [MOV(@8b565331@[5],@c7ddefd3@.Mailbox.Class2AcyclicRead.In.DataSize) ,MOV(@8b565331@[10],@c7ddefd3@.Mailbox.Class2AcyclicRead.In.C_REF) ,COP(@8b565331@[11],@c7ddefd3@.Mailbox.Class2AcyclicRead.In.Index,2) ,COP(@8b565331@[12],@c7ddefd3@.Mailbox.Class2AcyclicRead.In.Length,2) ,COP(@8b565331@[14],@c7ddefd3@.Mailbox.Class2AcyclicRead.In.ErrorDecode,1) ,COP(@8b565331@[15],@c7ddefd3@.Mailbox.Class2AcyclicRead.In.ErrorCode2,2) ,MOV(@8b565331@[16],@c7ddefd3@.Mailbox.Class2AcyclicRead.In.ExtendedFaultInfo) ,MOV(@8b565331@[17],@c7ddefd3@.Mailbox.Class2AcyclicRead.In.FaultInformation) ,COP(@8b565331@[18],@c7ddefd3@.Mailbox.Class2AcyclicRead.In.Data[0],88) ,LEQ(@c7ddefd3@.Mailbox.Class2AcyclicRead.In.DataSize,88) OTU(@c7ddefd3@.Util.FinishClass2AcyclicRead) ] ,EQU(101,@c7ddefd3@.BP.LastRead) [SUB(@c7ddefd3@.Mailbox.Class2AcyclicRead.In.DataSize,88,@c7ddefd3@.Mailbox.Class2AcyclicRead.In.DataSize) ,COP(@8b565331@[2],@c7ddefd3@.Mailbox.Class2AcyclicRead.In.Data[208],120) ,LEQ(@c7ddefd3@.Mailbox.Class2AcyclicRead.In.DataSize,120) OTU(@c7ddefd3@.Util.FinishClass2AcyclicRead) ] ,EQU(102,@c7ddefd3@.BP.LastRead) [COP(@8b565331@[2],@c7ddefd3@.Mailbox.Class2AcyclicRead.In.Data[208],48) ,OTU(@c7ddefd3@.Util.FinishClass2AcyclicRead) ] ] ,XIC(@c7ddefd3@.Util.FinishClass2AcyclicWrite) [EQU(100,@c7ddefd3@.BP.LastRead) EQU(@8b565331@[4],40) [MOV(@8b565331@[5],@c7ddefd3@.Mailbox.Class2AcyclicWrite.In.ByteCount) ,MOV(@8b565331@[10],@c7ddefd3@.Mailbox.Class2AcyclicWrite.In.C_REF) ,COP(@8b565331@[11],@c7ddefd3@.Mailbox.Class2AcyclicWrite.In.Index,2) ,COP(@8b565331@[12],@c7ddefd3@.Mailbox.Class2AcyclicWrite.In.Length,1) ,COP(@8b565331@[14],@c7ddefd3@.Mailbox.Class2AcyclicWrite.In.ErrorDecode,1) ,COP(@8b565331@[15],@c7ddefd3@.Mailbox.Class2AcyclicWrite.In.ErrorCode2,2) ,MOV(@8b565331@[16],@c7ddefd3@.Mailbox.Class2AcyclicWrite.In.ExtendedFaultInfo) ,MOV(@8b565331@[17],@c7ddefd3@.Mailbox.Class2AcyclicWrite.In.FaultInformation) ,COP(@8b565331@[18],@c7ddefd3@.Mailbox.Class2AcyclicWrite.In.Data[0],88) ,LEQ(@c7ddefd3@.Mailbox.Class2AcyclicWrite.In.ByteCount,88) OTU(@c7ddefd3@.Util.FinishClass2AcyclicWrite) ,GRT(@c7ddefd3@.Mailbox.Class2AcyclicWrite.In.ByteCount,88) OTL(@c7ddefd3@.Util.Finishmailboxreading) ] ,EQU(101,@c7ddefd3@.BP.LastRead) XIC(@c7ddefd3@.Util.Finishmailboxreading) [LES(@c7ddefd3@.Mailbox.Class2AcyclicWrite.In.ByteCount,120) [COP(@8b565331@[2],@c7ddefd3@.Mailbox.Class2AcyclicWrite.In.Data[88],120) ,OTU(@c7ddefd3@.Util.FinishClass2AcyclicWrite) ,OTU(@c7ddefd3@.Util.Finishmailboxreading) ,OTU(@c7ddefd3@.Util.Class2AcyclicWrite101) ] ,GRT(@c7ddefd3@.Mailbox.Class2AcyclicWrite.In.ByteCount,120) OTL(@c7ddefd3@.Util.Finishmailboxreading) ] ,EQU(102,@c7ddefd3@.BP.LastRead) XIC(@c7ddefd3@.Util.Finishmailboxreading) [COP(@8b565331@[2],@c7ddefd3@.Mailbox.Class2AcyclicWrite.In.Data[208],36) ,OTU(@c7ddefd3@.Util.FinishClass2AcyclicWrite) ,OTU(@c7ddefd3@.Util.Finishmailboxreading) ] ] ] ,LIM(200,@c7ddefd3@.BP.LastRead,202) [EQU(@c7ddefd3@.BP.LastRead,200) [MOV(@8b565331@[5],@c7ddefd3@.Mailbox.Alarm.ByteCount) ,COP(@8b565331@[10],@c7ddefd3@.Mailbox.Alarm.SlotNumber,2) ,COP(@8b565331@[11],@c7ddefd3@.Mailbox.Alarm.AlarmSpecAck,2) ,COP(@8b565331@[12],@c7ddefd3@.Mailbox.Alarm.ExtDiag,2) ,MOV(@8b565331@[17],@c7ddefd3@.Mailbox.Alarm.FaultInformation) ,COP(@8b565331@[18],@c7ddefd3@.Mailbox.Alarm.Data[0],88) ] ,EQU(@c7ddefd3@.BP.LastRead,201) COP(@8b565331@[2],@c7ddefd3@.Mailbox.Alarm.Data[88],120) ,EQU(@c7ddefd3@.BP.LastRead,202) COP(@8b565331@[2],@c7ddefd3@.Mailbox.Alarm.Data[208],48) ] ,EQU(@8b565331@[0],@c7ddefd3@.BP.LastRead) [MOV(@8b565331@[1],@c7ddefd3@.BP.LastWrite) ,XIC(@c7ddefd3@.MailboxCommand.StopMode) [MOV(100,@c7ddefd3@.BP.LastWrite) ,MOV(2,@7f34e890@[1]) ,MOV(16386,@7f34e890@[2]) ,MOV(2,@7f34e890@[3]) ,MOV(0,@7f34e890@[4]) ,MOV(1,@7f34e890@[5]) ,MOV(1,@7f34e890@[6]) ,MOV(0,@7f34e890@[7]) ,MOV(0,@7f34e890@[8]) ,MOV(16384,@7f34e890@[9]) ] ,XIC(@c7ddefd3@.MailboxCommand.OperateMode) [MOV(100,@c7ddefd3@.BP.LastWrite) ,MOV(1,@7f34e890@[1]) ,MOV(16386,@7f34e890@[2]) ,MOV(2,@7f34e890@[3]) ,MOV(0,@7f34e890@[4]) ,MOV(1,@7f34e890@[5]) ,MOV(1,@7f34e890@[6]) ,MOV(0,@7f34e890@[7]) ,MOV(0,@7f34e890@[8]) ,MOV(-16384,@7f34e890@[9]) ] ,XIC(@c7ddefd3@.MailboxCommand.ClearMode) [MOV(100,@c7ddefd3@.BP.LastWrite) ,MOV(3,@7f34e890@[1]) ,MOV(16386,@7f34e890@[2]) ,MOV(2,@7f34e890@[3]) ,MOV(0,@7f34e890@[4]) ,MOV(1,@7f34e890@[5]) ,MOV(1,@7f34e890@[6]) ,MOV(0,@7f34e890@[7]) ,MOV(0,@7f34e890@[8]) ,MOV(-32768,@7f34e890@[9]) ] ,XIC(@c7ddefd3@.MailboxCommand.GetLiveList) XIO(@c7ddefd3@.Util.Finishgetlivelist) [MOV(100,@c7ddefd3@.BP.LastWrite) ,MOV(4,@7f34e890@[1]) ,MOV(16386,@7f34e890@[2]) ,MOV(24,@7f34e890@[3]) ,MOV(0,@7f34e890@[4]) ,MOV(1,@7f34e890@[5]) ,MOV(1,@7f34e890@[6]) ,MOV(0,@7f34e890@[7]) ,MOV(0,@7f34e890@[8]) ,OTU(@c7ddefd3@.MailboxCommand.GetLiveList) ,OTL(@c7ddefd3@.Util.Finishgetlivelist) ] ,XIC(@c7ddefd3@.MailboxCommand.GetSlaveConfig) XIO(@c7ddefd3@.Util.FinishgetSlaveconfig) [MOV(100,@c7ddefd3@.BP.LastWrite) ,MOV(5,@7f34e890@[1]) ,MOV(16386,@7f34e890@[2]) ,MOV(5,@7f34e890@[3]) ,MOV(0,@7f34e890@[4]) ,MOV(1,@7f34e890@[5]) ,MOV(1,@7f34e890@[6]) ,MOV(0,@7f34e890@[7]) ,MOV(0,@7f34e890@[8]) ,SWPB(@c7ddefd3@.Mailbox.GetSlaveConfig.Out.SlaveAddress,REVERSE,@c7ddefd3@.Util.ByteSwapUtil) ,MOV(@c7ddefd3@.Util.ByteSwapUtil,@7f34e890@[9]) ,OTU(@c7ddefd3@.MailboxCommand.GetSlaveConfig) ,OTL(@c7ddefd3@.Util.FinishgetSlaveconfig) ] ,XIC(@c7ddefd3@.MailboxCommand.SetSlaveMode) [MOV(100,@c7ddefd3@.BP.LastWrite) ,MOV(6,@7f34e890@[1]) ,MOV(16386,@7f34e890@[2]) ,MOV(3,@7f34e890@[3]) ,MOV(0,@7f34e890@[4]) ,MOV(1,@7f34e890@[5]) ,MOV(1,@7f34e890@[6]) ,MOV(0,@7f34e890@[7]) ,MOV(0,@7f34e890@[8]) ,COP(@c7ddefd3@.Mailbox.SetSlaveMode.Out.GroupSelect,@7f34e890@[9],1) ,COP(@c7ddefd3@.Mailbox.SetSlaveMode.Out.ControlCommand,@c7ddefd3@.Util.TempInt,1) ,SWPB(@c7ddefd3@.Util.TempInt,REVERSE,@c7ddefd3@.Util.ByteSwapUtil) ,MOV(@c7ddefd3@.Util.ByteSwapUtil,@7f34e890@[10]) ] ,XIC(@c7ddefd3@.MailboxCommand.GetSlaveDiagnostics) XIO(@c7ddefd3@.Util.FinishgetSlaveDiagnost) [MOV(100,@c7ddefd3@.BP.LastWrite) ,MOV(7,@7f34e890@[1]) ,MOV(16386,@7f34e890@[2]) ,MOV(4,@7f34e890@[3]) ,MOV(0,@7f34e890@[4]) ,MOV(1,@7f34e890@[5]) ,MOV(1,@7f34e890@[6]) ,MOV(0,@7f34e890@[7]) ,MOV(0,@7f34e890@[8]) ,COP(@c7ddefd3@.Mailbox.GetSlaveDiagnostics.Out.RequestType,@7f34e890@[9],1) ,OTU(@c7ddefd3@.MailboxCommand.GetSlaveDiagnostics) ,OTL(@c7ddefd3@.Util.FinishgetSlaveDiagnost) ] ,XIC(@c7ddefd3@.Util.SetSlaveAddress102) [MOV(102,@c7ddefd3@.BP.LastWrite) ,COP(@c7ddefd3@.Mailbox.SetSlaveAddress.In.MessageDataByte[208],@7f34e890@[1],24) ,OTU(@c7ddefd3@.Util.SetSlaveAddress102) ] ,XIC(@c7ddefd3@.Util.SetSlaveAddress101) [MOV(101,@c7ddefd3@.BP.LastWrite) ,COP(@c7ddefd3@.Mailbox.SetSlaveAddress.In.MessageDataByte[88],@7f34e890@[1],60) ,GRT(@c7ddefd3@.Mailbox.SetSlaveAddress.Out.ByteCount,120) [OTL(@c7ddefd3@.Util.SetSlaveAddress102) ,OTL(@c7ddefd3@.Util.Finishmailboxreading) ] ,OTU(@c7ddefd3@.Util.SetSlaveAddress101) ] ,XIC(@c7ddefd3@.MailboxCommand.SetSlaveAddress) XIO(@c7ddefd3@.Util.FinishSetSlaveAddr) [MOV(100,@c7ddefd3@.BP.LastWrite) ,MOV(8,@7f34e890@[1]) ,MOV(16386,@7f34e890@[2]) ,MOV(6,@7f34e890@[3]) ,MOV(@c7ddefd3@.Mailbox.SetSlaveAddress.Out.ByteCount,@7f34e890@[4]) ,MOV(1,@7f34e890@[5]) ,MOV(1,@7f34e890@[6]) ,MOV(0,@7f34e890@[7]) ,MOV(0,@7f34e890@[8]) ,COP(@c7ddefd3@.Mailbox.SetSlaveAddress.Out.NewSlaveAddress,@7f34e890@[9],1) ,MOV(@c7ddefd3@.Mailbox.SetSlaveAddress.Out.SlaveIdentNumber,@7f34e890@[10]) ,SWPB(@c7ddefd3@.Mailbox.SetSlaveAddress.Out.No_add_Chg,REVERSE,@c7ddefd3@.Util.ByteSwapUtil) ,MOV(@c7ddefd3@.Util.ByteSwapUtil,@7f34e890@[11]) ,COP(@c7ddefd3@.Mailbox.SetSlaveAddress.Out.MessageDataByte[0],@7f34e890@[17],42) ,OTU(@c7ddefd3@.MailboxCommand.SetSlaveAddress) ,OTL(@c7ddefd3@.Util.FinishSetSlaveAddr) ] ,XIC(@c7ddefd3@.Util.FinishStartStopSlaves) EQU(@c7ddefd3@.BP.LastWrite,101) [MOV(101,@c7ddefd3@.BP.LastWrite) ,COP(@c7ddefd3@.Mailbox.StartStopSlaves.Out.SlaveNumber[88],@7f34e890@[1],19) ] ,XIC(@c7ddefd3@.MailboxCommand.StartSlaves) XIO(@c7ddefd3@.Util.FinishStartStopSlaves) [MOV(100,@c7ddefd3@.BP.LastWrite) ,MOV(16,@7f34e890@[1]) ,MOV(16386,@7f34e890@[2]) ,MOV(11,@7f34e890@[3]) ,MOV(126,@7f34e890@[4]) ,MOV(1,@7f34e890@[5]) ,MOV(1,@7f34e890@[6]) ,MOV(0,@7f34e890@[7]) ,MOV(0,@7f34e890@[8]) ,MOV(0,@7f34e890@[9]) ,MOV(0,@7f34e890@[10]) ,MOV(0,@7f34e890@[11]) ,MOV(0,@7f34e890@[12]) ,MOV(0,@7f34e890@[13]) ,MOV(0,@7f34e890@[14]) ,MOV(0,@7f34e890@[15]) ,MOV(0,@7f34e890@[16]) ,COP(@c7ddefd3@.Mailbox.StartStopSlaves.Out.SlaveNumber[0],@7f34e890@[17],44) ,OTU(@c7ddefd3@.MailboxCommand.StartSlaves) ,OTL(@c7ddefd3@.Util.FinishStartStopSlaves) ] ,XIC(@c7ddefd3@.MailboxCommand.StopSlaves) XIO(@c7ddefd3@.Util.FinishStartStopSlaves) [MOV(100,@c7ddefd3@.BP.LastWrite) ,MOV(17,@7f34e890@[1]) ,MOV(16386,@7f34e890@[2]) ,MOV(12,@7f34e890@[3]) ,MOV(126,@7f34e890@[4]) ,MOV(1,@7f34e890@[5]) ,MOV(1,@7f34e890@[6]) ,MOV(0,@7f34e890@[7]) ,MOV(0,@7f34e890@[8]) ,MOV(0,@7f34e890@[9]) ,MOV(0,@7f34e890@[10]) ,MOV(0,@7f34e890@[11]) ,MOV(0,@7f34e890@[12]) ,MOV(0,@7f34e890@[13]) ,MOV(0,@7f34e890@[14]) ,MOV(0,@7f34e890@[15]) ,MOV(0,@7f34e890@[16]) ,COP(@c7ddefd3@.Mailbox.StartStopSlaves.Out.SlaveNumber[0],@7f34e890@[17],44) ,OTU(@c7ddefd3@.MailboxCommand.StopSlaves) ,OTL(@c7ddefd3@.Util.FinishStartStopSlaves) ] ,XIC(@c7ddefd3@.MailboxCommand.Class1AcyclicRead) XIO(@c7ddefd3@.Util.FinishClass1AcyclicRead) [MOV(100,@c7ddefd3@.BP.LastWrite) ,MOV(9,@7f34e890@[1]) ,MOV(16386,@7f34e890@[2]) ,MOV(32,@7f34e890@[3]) ,COP(@c7ddefd3@.Mailbox.Class1AcyclicRead.Out.DataSize,@c7ddefd3@.Mailbox.Class1AcyclicRead.Out.Length,1) ,MOV(0,@7f34e890@[4]) ,MOV(1,@7f34e890@[5]) ,MOV(1,@7f34e890@[6]) ,MOV(0,@7f34e890@[7]) ,MOV(0,@7f34e890@[8]) ,COP(@c7ddefd3@.Mailbox.Class1AcyclicRead.Out.SlotNumber,@7f34e890@[9],1) ,COP(@c7ddefd3@.Mailbox.Class1AcyclicRead.Out.Length,@7f34e890@[10],1) ,OTU(@c7ddefd3@.MailboxCommand.Class1AcyclicRead) ,OTL(@c7ddefd3@.Util.FinishClass1AcyclicRead) ] ,XIC(@c7ddefd3@.Util.Class1AcyclicWrite102) [MOV(102,@c7ddefd3@.BP.LastWrite) ,COP(@c7ddefd3@.Mailbox.Class1AcyclicWrite.Out.Data[208],@7f34e890@[1],24) ,OTU(@c7ddefd3@.Util.Class1AcyclicWrite102) ] ,XIC(@c7ddefd3@.Util.Class1AcyclicWrite101) [MOV(101,@c7ddefd3@.BP.LastWrite) ,COP(@c7ddefd3@.Mailbox.Class1AcyclicWrite.Out.Data[88],@7f34e890@[1],60) ,GRT(@c7ddefd3@.Util.TempInt2,120) OTL(@c7ddefd3@.Util.Class1AcyclicWrite102) ,OTU(@c7ddefd3@.Util.Class1AcyclicWrite101) ] ,XIC(@c7ddefd3@.MailboxCommand.Class1AcyclicWrite) XIO(@c7ddefd3@.Util.FinishClass1AcyclicWrite) [MOV(100,@c7ddefd3@.BP.LastWrite) ,MOV(10,@7f34e890@[1]) ,MOV(16386,@7f34e890@[2]) ,MOV(33,@7f34e890@[3]) ,COP(@c7ddefd3@.Mailbox.Class1AcyclicWrite.Out.DataSize,@c7ddefd3@.Mailbox.Class1AcyclicWrite.Out.Length,1) ,COP(@c7ddefd3@.Mailbox.Class1AcyclicWrite.Out.DataSize,@c7ddefd3@.Util.TempInt2,1) ,MOV(@c7ddefd3@.Mailbox.Class1AcyclicWrite.Out.DataSize,@7f34e890@[4]) ,MOV(1,@7f34e890@[5]) ,MOV(1,@7f34e890@[6]) ,MOV(0,@7f34e890@[7]) ,MOV(0,@7f34e890@[8]) ,COP(@c7ddefd3@.Mailbox.Class1AcyclicWrite.Out.SlotNumber,@7f34e890@[9],1) ,COP(@c7ddefd3@.Mailbox.Class1AcyclicWrite.Out.Length,@7f34e890@[10],1) ,COP(@c7ddefd3@.Mailbox.Class1AcyclicWrite.Out.Data[0],@7f34e890@[17],44) ,GRT(@c7ddefd3@.Util.TempInt2,88) [SUB(@c7ddefd3@.Util.TempInt2,88,@c7ddefd3@.Util.TempInt2) ,OTL(@c7ddefd3@.Util.Class1AcyclicWrite101) ] ,OTL(@c7ddefd3@.Util.FinishClass1AcyclicWrite) ,OTU(@c7ddefd3@.MailboxCommand.Class1AcyclicWrite) ] ,XIC(@c7ddefd3@.MailboxCommand.InitiateConnection) [MOV(100,@c7ddefd3@.BP.LastWrite) ,MOV(11,@7f34e890@[1]) ,MOV(16386,@7f34e890@[2]) ,MOV(37,@7f34e890@[3]) ,MOV(0,@7f34e890@[4]) ,MOV(1,@7f34e890@[5]) ,MOV(1,@7f34e890@[6]) ,MOV(0,@7f34e890@[7]) ,MOV(0,@7f34e890@[8]) ,MOV(@c7ddefd3@.Mailbox.InitiateConnection.Out.C_REF,@7f34e890@[9]) ,SWPB(@c7ddefd3@.Mailbox.InitiateConnection.Out.SlaveAddress,REVERSE,@c7ddefd3@.Util.ByteSwapUtil) ,MOV(@c7ddefd3@.Util.ByteSwapUtil,@7f34e890@[10]) ,OTU(@c7ddefd3@.MailboxCommand.InitiateConnection) ] ,XIC(@c7ddefd3@.MailboxCommand.AbortConnection) [MOV(100,@c7ddefd3@.BP.LastWrite) ,MOV(12,@7f34e890@[1]) ,MOV(16386,@7f34e890@[2]) ,MOV(38,@7f34e890@[3]) ,MOV(0,@7f34e890@[4]) ,MOV(1,@7f34e890@[5]) ,MOV(1,@7f34e890@[6]) ,MOV(0,@7f34e890@[7]) ,MOV(0,@7f34e890@[8]) ,MOV(@c7ddefd3@.Mailbox.AbortConnection.Out.C_REF,@7f34e890@[9]) ,COP(@c7ddefd3@.Mailbox.AbortConnection.Out.ReasonCode,@7f34e890@[10],1) ,OTU(@c7ddefd3@.MailboxCommand.AbortConnection) ] ,XIC(@c7ddefd3@.MailboxCommand.Class2AcyclicRead) XIO(@c7ddefd3@.Util.FinishClass2AcyclicRead) [MOV(100,@c7ddefd3@.BP.LastWrite) ,MOV(9,@7f34e890@[1]) ,MOV(16386,@7f34e890@[2]) ,MOV(39,@7f34e890@[3]) ,MOV(0,@7f34e890@[4]) ,MOV(1,@7f34e890@[5]) ,MOV(1,@7f34e890@[6]) ,MOV(0,@7f34e890@[7]) ,MOV(0,@7f34e890@[8]) ,MOV(@c7ddefd3@.Mailbox.Class2AcyclicRead.Out.C_REF,@7f34e890@[9]) ,COP(@c7ddefd3@.Mailbox.Class2AcyclicRead.Out.Index,@7f34e890@[10],1) ,SWPB(@c7ddefd3@.Mailbox.Class2AcyclicRead.Out.Length,REVERSE,@c7ddefd3@.Util.ByteSwapUtil) ,MOV(@c7ddefd3@.Util.ByteSwapUtil,@7f34e890@[11]) ,OTU(@c7ddefd3@.MailboxCommand.Class2AcyclicRead) ,OTL(@c7ddefd3@.Util.FinishClass2AcyclicRead) ] ,XIC(@c7ddefd3@.Util.Class2AcyclicWrite102) [MOV(102,@c7ddefd3@.BP.LastWrite) ,COP(@c7ddefd3@.Mailbox.Class2AcyclicWrite.Out.Data[208],@7f34e890@[1],24) ,OTU(@c7ddefd3@.Util.Class2AcyclicWrite102) ] ,XIC(@c7ddefd3@.Util.Class2AcyclicWrite101) [MOV(101,@c7ddefd3@.BP.LastWrite) ,COP(@c7ddefd3@.Mailbox.Class2AcyclicWrite.Out.Data[88],@7f34e890@[1],60) ,GRT(@c7ddefd3@.Util.TempInt2,120) OTL(@c7ddefd3@.Util.Class2AcyclicWrite102) ,OTU(@c7ddefd3@.Util.Class2AcyclicWrite101) ] ,XIC(@c7ddefd3@.MailboxCommand.Class2AcyclicWrite) XIO(@c7ddefd3@.Util.FinishClass2AcyclicWrite) [MOV(100,@c7ddefd3@.BP.LastWrite) ,MOV(10,@7f34e890@[1]) ,MOV(16386,@7f34e890@[2]) ,MOV(40,@7f34e890@[3]) ,COP(@c7ddefd3@.Mailbox.Class2AcyclicWrite.Out.DataSize,@c7ddefd3@.Mailbox.Class2AcyclicWrite.Out.Length,1) ,COP(@c7ddefd3@.Mailbox.Class2AcyclicWrite.Out.DataSize,@c7ddefd3@.Util.TempInt2,1) ,MOV(@c7ddefd3@.Mailbox.Class2AcyclicWrite.Out.DataSize,@7f34e890@[4]) ,MOV(1,@7f34e890@[5]) ,MOV(1,@7f34e890@[6]) ,MOV(0,@7f34e890@[7]) ,MOV(0,@7f34e890@[8]) ,MOV(@c7ddefd3@.Mailbox.Class2AcyclicWrite.Out.C_REF,@7f34e890@[9]) ,COP(@c7ddefd3@.Mailbox.Class2AcyclicWrite.Out.Index,@7f34e890@[10],1) ,SWPB(@c7ddefd3@.Mailbox.Class2AcyclicWrite.Out.Length,REVERSE,@c7ddefd3@.Util.ByteSwapUtil) ,MOV(@c7ddefd3@.Util.ByteSwapUtil,@7f34e890@[11]) ,COP(@c7ddefd3@.Mailbox.Class2AcyclicWrite.Out.Data[0],@7f34e890@[17],44) ,GRT(@c7ddefd3@.Util.TempInt2,88) [SUB(@c7ddefd3@.Util.TempInt2,88,@c7ddefd3@.Util.TempInt2) ,OTL(@c7ddefd3@.Util.Class2AcyclicWrite101) ] ,OTL(@c7ddefd3@.Util.FinishClass2AcyclicWrite) ,OTU(@c7ddefd3@.MailboxCommand.Class2AcyclicWrite) ] ,XIC(@c7ddefd3@.MailboxCommand.SynchCRC) [MOV(@c7ddefd3@.CRC.In.ProfibusCRC,@c7ddefd3@.CRC.Out.ProfibusCRC) ,MOV(@c7ddefd3@.CRC.In.ModuleCRC,@c7ddefd3@.CRC.Out.ModuleCRC) ,OTU(@c7ddefd3@.MailboxCommand.SynchCRC) ] ] ,LIM(1,@c7ddefd3@.BP.LastWrite,16) [CPT(@c7ddefd3@.BP.BlockIndex,(@c7ddefd3@.BP.LastWrite-1)*100) ,LIM(1,@c7ddefd3@.BP.LastWrite,15) COP(@c7ddefd3@.Output[@c7ddefd3@.BP.BlockIndex],@7f34e890@[1],50) ,EQU(@c7ddefd3@.BP.LastWrite,16) COP(@c7ddefd3@.Output[1500],@7f34e890@[1],36) ,COP(@c7ddefd3@.MailboxControl.Out_Last_Out_MB,@7f34e890@[51],2) ,COP(@c7ddefd3@.CRC.Out.ProfibusCRC,@7f34e890@[54],4) ] ,MOV(@c7ddefd3@.BP.LastWrite,@7f34e890@[0]) ];
END_ROUTINE
END_ADD_ON_INSTRUCTION

VAR_GLOBAL   (* controller tags *)
   AOI69PDPMV1_60 : AOI69PDPMV1_60;
   Local:1:I : AB:1769_MODULE_INT_128Bytes:I:0;
   Local:1:O : AB:1769_MODULE_INT_122Bytes:O:0;
   MVI69PDPMV1 : PDPMV1_ModuleDef;
END_VAR

PROGRAM MainProgram

ROUTINE MainRoutine   (* ladder *)
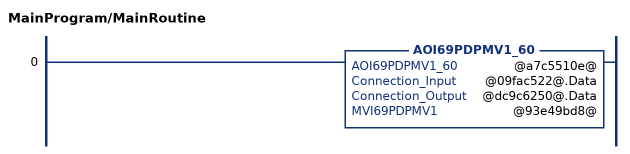
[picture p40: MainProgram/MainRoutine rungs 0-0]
   0: AOI69PDPMV1_60(@a7c5510e@,@09fac522@.Data,@dc9c6250@.Data,@93e49bd8@);
END_ROUTINE
END_PROGRAM
